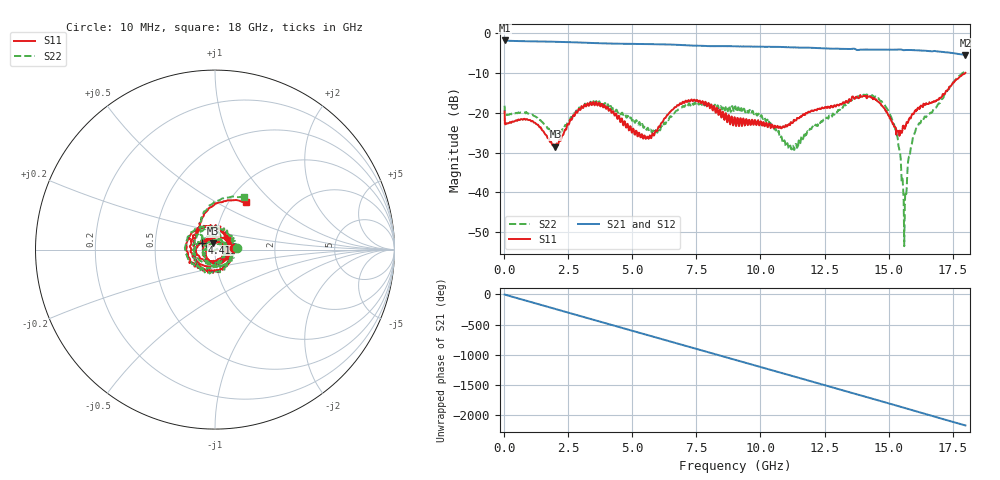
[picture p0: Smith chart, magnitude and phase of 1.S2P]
!Agilent Technologies,E5071C,MY46316741,A.11.02
!Date: Tue Sep 22 10:33:23 2020
!Data & Calibration Information:
!Freq	S11:SOLT4(ON)	S21:SOLT4(ON)	S12:SOLT4(ON)	S22:SOLT4(ON)
!PortZ  Port1:50+j0  Port2:50+j0
!Above PortZ is port z conversion or system Z0 setting when saving the data.
!When reading, reference impedance value at option line is always used.
# Hz S dB R 50
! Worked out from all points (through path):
!   1561 points, 10 MHz to 18 GHz, reference 50 ohm
!   highest |S21| = -1.89 dB at 10 MHz (marker M1); lowest = -5.5 dB at 18 GHz (marker M2)
!   group delay of S21, straight-line fit = 335 ps
!   lowest |S11| = -28.5 dB at 1.994 GHz (marker M3), VSWR 1.08, Z = 48.7 + j3.49 ohm
!   |S11| at or under -10 dB: start of sweep to end of sweep
!   |S22| runs from -53.5 to -9.5 dB; largest |S21 - S12| = 0.02
!   S11 on the Smith chart (normalised r, x): 10 MHz: 1.23, +0.02; 4.415 GHz: 0.86, +0.07; 18 GHz: 1.19, +0.70
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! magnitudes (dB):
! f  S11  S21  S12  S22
! 10 MHz  -19.7  -1.9  -1.9  -18.3
! 1.14 GHz  -22.4  -2.1  -2.1  -20.8
! 1.994 GHz  -28.5  -2.2  -2.2  -25.4
! 3.02 GHz  -18.4  -2.4  -2.4  -18.3
! 3.643 GHz  -18.2  -2.6  -2.6  -17.7
! 4.415 GHz  -21.6  -2.7  -2.7  -19.8
! 5.476 GHz  -25.7  -2.8  -2.8  -23.4
! 6.007 GHz  -23.7  -2.9  -2.9  -24.2
! 6.687 GHz  -18.7  -3.0  -3.0  -19.7
! 7.356 GHz  -17.1  -3.2  -3.2  -17.8
! 9.005 GHz  -21.4  -3.4  -3.4  -18.5
! 10.1 GHz  -22.5  -3.5  -3.5  -21.6
! 11.16 GHz  -23.0  -3.6  -3.6  -28.2
! 12.01 GHz  -19.5  -3.7  -3.8  -23.7
! 13.98 GHz  -16.0  -4.2  -4.2  -15.7
! 15 GHz  -20.7  -4.2  -4.2  -19.8
! 15.38 GHz  -24.7  -4.2  -4.3  -28.0
! 15.56 GHz  -23.4  -4.3  -4.1  -37.3
! 15.64 GHz  -24.0  -4.3  -4.2  -43.5
! 15.82 GHz  -21.3  -4.3  -4.3  -30.8
! 16.1 GHz  -19.4  -4.4  -4.4  -23.8
! 18 GHz  -10.0  -5.5  -5.6  -9.5
